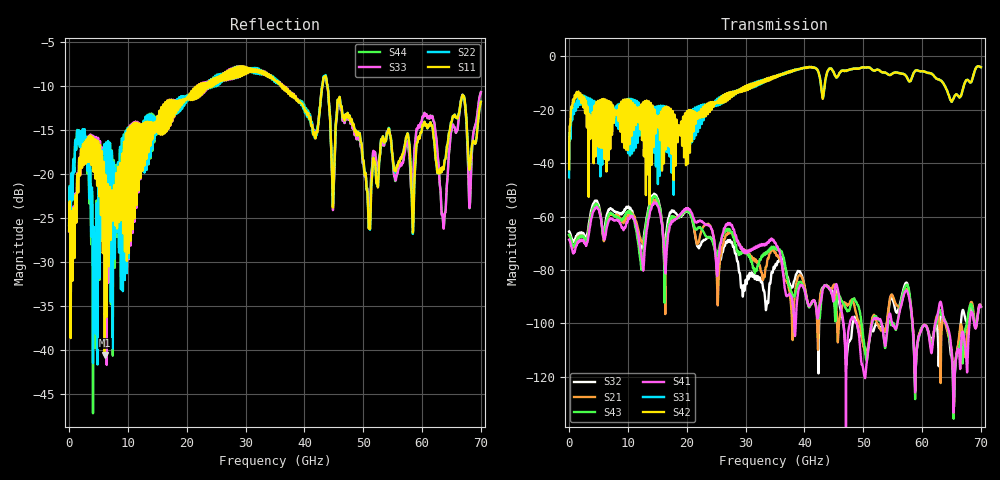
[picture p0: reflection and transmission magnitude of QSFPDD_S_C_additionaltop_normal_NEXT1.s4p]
! AWR Design Environment (8415) Thu Dec 20 13:40:35 2018
! Document = 'CHANNEL TEST'
! nPorts: 4, nXvals: 7001
# HZ S DB R 50
!Freq DBS11 AngS11 DBS12 AngS12 DBS13 AngS13 DBS14 AngS14
!	DBS21 AngS21 DBS22 AngS22 DBS23 AngS23 DBS24 AngS24
!	DBS31 AngS31 DBS32 AngS32 DBS33 AngS33 DBS34 AngS34
!	DBS41 AngS41 DBS42 AngS42 DBS43 AngS43 DBS44 AngS44
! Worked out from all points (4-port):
!   7000 points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, 10 MHz to 70 GHz, reference 50 ohm
!   strongest paths, dB at 10 MHz, 17.51 GHz, 35.01 GHz, 52.51 GHz, 70 GHz:
!     S42: -42.2, -24.0, -7.5, -5.0, -4.0
!     S31: -45.3, -23.9, -7.5, -5.0, -4.0
!     S41: -68.6, -61.5, -69.8, -98.2, -93.8
!     S43: -66.8, -59.8, -71.9, -98.2, -93.6
!     S21: -66.9, -60.1, -73.6, -100.3, -93.8
!     S32: -65.5, -57.7, -78.8, -100.6, -93.6
!   lowest |S11| = -40.5 dB at 6.06 GHz (marker M1), VSWR 1.02, Z = 49.4 + j0.738 ohm
!   |S11| at or under -10 dB: start of sweep to 21.77 GHz; 36.5 GHz to 43.04 GHz (6.538 GHz wide, 16.4 % of centre); 43.94 GHz to end of sweep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
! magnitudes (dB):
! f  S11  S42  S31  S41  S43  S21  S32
! 10 MHz  -26.5  -42.2  -45.3  -68.6  -66.8  -66.9  -65.5
! 1.29 GHz  -23.5  -13.3  -16.8  -70.7  -69.0  -68.7  -67.2
! 6.06 GHz  -40.5  -29.3  -18.8  -68.3  -65.7  -67.7  -64.1
! 12.3 GHz  -14.3  -19.5  -24.4  -75.0  -79.7  -69.3  -72.2
! 14.54 GHz  -15.2  -20.0  -19.9  -54.8  -52.5  -53.8  -51.6
! 29.19 GHz  -7.7  -12.1  -12.2  -72.0  -74.1  -71.9  -85.5
! 70 GHz  -11.8  -4.0  -4.0  -93.8  -93.6  -93.8  -93.6
